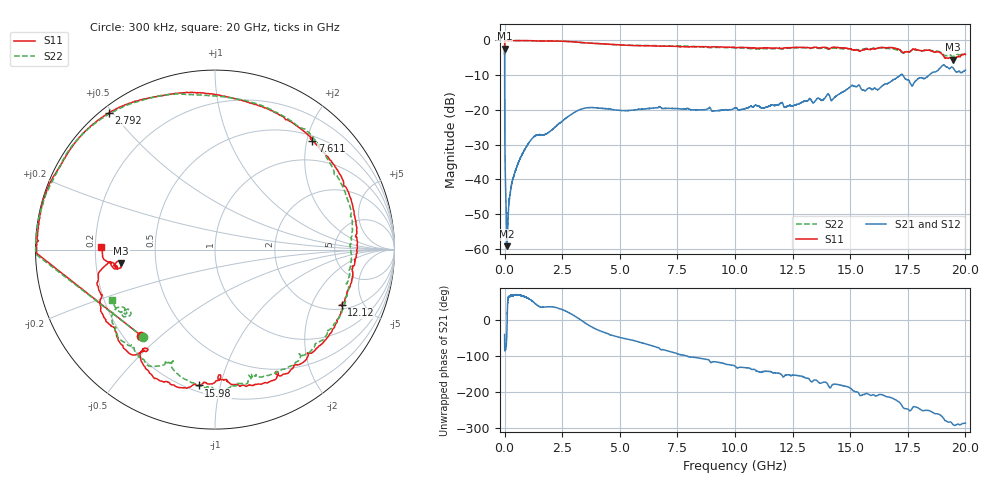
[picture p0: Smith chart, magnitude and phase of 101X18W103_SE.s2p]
!{101X18W103_SE}
!Johanson Technology Inc.
!www.johansontechnology.com
!Test Board Conditions:
!Substrate Type  RO4350B
!Substrate Thickness  21 mil
!Substrate Dk  3.66
!TL Type: GCPW
!TL Trace Width  40 mil
!TL Gap  20 mil
!PART MODE SINGLE ENDED (AKA BYPASS)
!DUT TOPOLOGY	SERIES-SHUNT
!Mounting Pad LxW  120x40 mil
! Created Wed Oct 27 11:11:12 2021
# hz S ma R 50
! 2 Port Network Data from SP1.SP block
! freq  magS11  angS11  magS21  angS21  magS12  angS12  magS22  angS22
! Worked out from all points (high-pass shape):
!   20001 points, 300 kHz to 20 GHz, reference 50 ohm
!   highest |S21| = -2.32 dB at 300 kHz (marker M1); lowest = -59.2 dB at 107.3 MHz (marker M2)
!   |S21| within 3 dB of the highest: start of sweep to 632.9 kHz
!   lowest |S11| = -5.5 dB at 19.45 GHz (marker M3), VSWR 3.24, Z = 15.5 - j3.24 ohm
!   |S11| at or under -10 dB: nowhere
!   |S22| runs from -4.7 to 0.0 dB; largest |S21 - S12| = 0.011
!   S11 on the Smith chart (normalised r, x): 300 kHz: 0.27, -0.43; 2.792 GHz: 0.02, +0.49; 7.611 GHz: 0.59, +2.10; 12.12 GHz: 2.22, -3.39; 15.98 GHz: 0.24, -0.86; 20 GHz: 0.23, +0.01
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300000  0.6316 -130.6  0.7657 -39.0  0.769 -39.5  0.6302 -129.4
1.073e8  0.9939 178.2  0.001092 -10.0  0.001171 -10.4  0.9998 178.2
1.683e8  0.9904 176.9  0.003658 66.7  0.003497 65.3  0.9998 177.0
2.843e8  0.9933 174.7  0.00774 70.6  0.007767 69.9  0.9992 175.0
4.743e8  0.993 171.2  0.01344 71.8  0.01348 71.6  0.9978 171.6
1.0433e9  0.9936 160.6  0.03319 61.1  0.03337 61.1  0.9901 161.3
2.7923e9  0.9651 127.8  0.08177 21.8  0.08218 21.7  0.9617 129.7
3.3343e9  0.9329 117.2  0.1028 0.2  0.103 0.1  0.9336 118.6
6.6673e9  0.8315 62.8  0.1081 -75.9  0.1084 -76.2  0.8413 68.1
7.6113e9  0.8126 48.2  0.1036 -95.4  0.1033 -95.2  0.8365 52.2
1.00003e10  0.7908 6.2  0.1074 -127.8  0.1082 -127.6  0.7805 14.5
1.21153e10  0.771 -23.7  0.112 -157.8  0.111 -157.8  0.7639 -14.5
1.33343e10  0.781 -48.3  0.1336 -171.7  0.1341 -171.2  0.7714 -36.1
1.50983e10  0.7344 -84.9  0.226 165.0  0.2251 164.3  0.7374 -72.1
1.59843e10  0.7625 -96.9  0.1975 152.4  0.1987 152.3  0.7685 -81.5
1.66673e10  0.7901 -111.3  0.2441 146.2  0.2419 148.1  0.7666 -95.3
1.72223e10  0.7005 -126.0  0.3238 124.5  0.3249 125.7  0.6826 -110.7
1.76983e10  0.7432 -127.7  0.2214 115.3  0.2234 114.9  0.7297 -117.0
1.84673e10  0.7167 -152.4  0.3252 106.8  0.328 106.6  0.7198 -139.3
1.90173e10  0.6189 -171.6  0.437 89.3  0.439 89.5  0.6407 -149.3
1.94523e10  0.5286 -171.8  0.407 69.4  0.4036 69.3  0.5856 -144.9
2e10  0.6294 178.5  0.3749 72.8  0.3745 71.9  0.6429 -154.2
